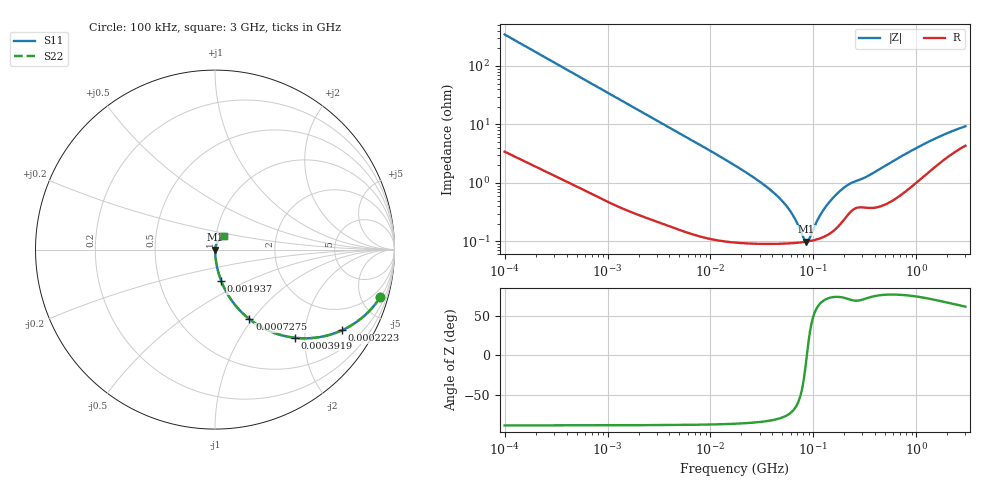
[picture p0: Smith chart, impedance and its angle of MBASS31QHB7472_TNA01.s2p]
! MBASS31QHB7472_TNA01  S-PARAMETER MODEL  ( Standard Model )
! Model Generated by TAIYO YUDEN Corporation (http://www.ty-top.com)
! Version 2.0
! TAIYO YUDEN Control No. 231201
! Copyright(c) 2013 TAIYO YUDEN CO.,LTD. All Rights Reserved.
! Product Description (link to TY-COMPAS)
! https://ds.yuden.co.jp/TYCOMPAS/or/detail?pn=MBASS31QHB7472KTNA01&u=M
! Products Name : Multilayer Ceramic Capacitors
! Characteristics :
!  Capacitance : 4700 [pF] , Rated Voltage : 630 [V] , TCC : X7R
!  Case Size : 3.2 x 1.6 / 0.126 x 0.063 [mm/inch] , Thickness : 1.15 / 0.045 [mm/inch]
!  (Conditions: Temperature = 25 [degC] , DC Bias Voltage = 0 [V])
! External Node Assignments :
!  1  o---| |---o  2
! GND o---------o GND
! Frequency Range : 100kHz  -  3GHz  [ 401 STEP ]
# MHZ S RI R 50
! Freq[MHz].  S11 Real  S11 Imag  S21 Real  S21 Imag  S12 Real  S12 Imag  S22 Real  S22 Imag
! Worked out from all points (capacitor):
!   401 points, 100 kHz to 3 GHz, reference 50 ohm
!   read as one part in series: C = 4.59 nF near 105.3 kHz
!   lowest |Z| = 99.3 mohm at 85.61 MHz (marker M1)
!   series resonance near 86.42 MHz, so ESL is about 740 pH
!   S11 on the Smith chart (normalised r, x): 100 kHz: 1.07, -6.93; 222.3 kHz: 1.03, -3.13; 391.9 kHz: 1.02, -1.78; 727.5 kHz: 1.01, -0.97; 1.937 MHz: 1.01, -0.36; 3 GHz: 1.09, +0.17
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0.1  0.9208 -0.2651  0.0792 0.2651  0.0792 0.2651  0.9208 -0.2651
0.222319  0.7082 -0.4491  0.2918 0.4491  0.2918 0.4491  0.7082 -0.4491
0.391939  0.4437 -0.4908  0.5563 0.4908  0.5563 0.4908  0.4437 -0.4908
0.562235  0.2823 -0.4439  0.7177 0.4439  0.7177 0.4439  0.2823 -0.4439
0.727522  0.1921 -0.3875  0.8079 0.3875  0.8079 0.3875  0.1921 -0.3875
1.127518  0.0921 -0.2824  0.9079 0.2824  0.9079 0.2824  0.0921 -0.2824
1.937191  0.0348 -0.1756  0.9652 0.1756  0.9652 0.1756  0.0348 -0.1756
3.161081  0.0145 -0.1103  0.9855 0.1103  0.9855 0.1103  0.0145 -0.1103
17.7727  0.00132 -0.0193  0.9987 0.0193  0.9987 0.0193  0.00132 -0.0193
32.98988  0.000992 -0.00929  0.999 0.00929  0.999 0.00929  0.000992 -0.00929
48.55934  0.000938 -0.00507  0.9991 0.00507  0.9991 0.00507  0.000938 -0.00507
62.83488  0.00094 -0.00271  0.9991 0.00271  0.9991 0.00271  0.00094 -0.00271
79.23846  0.000971 -0.000728  0.999 0.000728  0.999 0.000728  0.000971 -0.000728
85.60801  0.000989 -7.87e-05  0.999 7.87e-05  0.999 7.87e-05  0.000989 -7.87e-05
90.13636  0.001 0.000355  0.999 -0.000355  0.999 -0.000355  0.001 0.000355
97.38194  0.00103 0.00101  0.999 -0.00101  0.999 -0.00101  0.00103 0.00101
126.0104  0.0012 0.00329  0.9988 -0.00329  0.9988 -0.00329  0.0012 0.00329
180.7614  0.00197 0.00696  0.998 -0.00696  0.998 -0.00696  0.00197 0.00696
222.1509  0.00307 0.00898  0.9969 -0.00898  0.9969 -0.00898  0.00307 0.00898
547.5153  0.00506 0.021  0.9949 -0.021  0.9949 -0.021  0.00506 0.021
1420.79  0.0192 0.0495  0.9808 -0.0495  0.9808 -0.0495  0.0192 0.0495
3000  0.0475 0.0753  0.9525 -0.0753  0.9525 -0.0753  0.0475 0.0753
